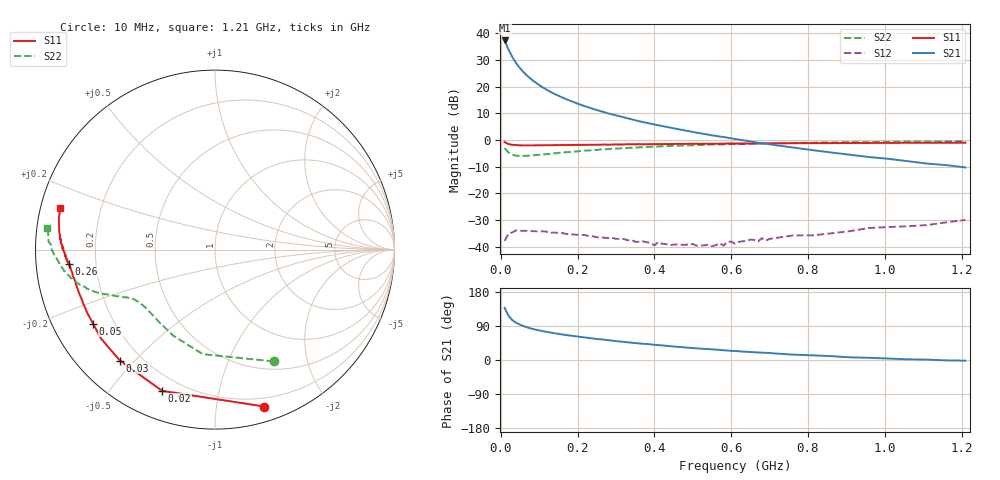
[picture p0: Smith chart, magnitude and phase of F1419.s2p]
! Fri Mar 13 15:57:41 1998
# MHZ  S  MA  R  50.0000
! SCATTERING PARAMETERS :
!  POLYFET RF DEVICES
!  F1419
!  S PARAMETERS
!  VDS=50V, IDQ=400mA
!FREQ  S11MAG S11ANG S21MAG S21ANG S12MAG S12ANG S22MAG S22ANG
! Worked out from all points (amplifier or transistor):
!   81 points, 10 MHz to 1.21 GHz, reference 50 ohm
!   highest |S21| = 37.3 dB at 10 MHz (marker M1)
!   |S21| within 3 dB of that: start of sweep to 18.98 MHz
!   unconditionally stable (mu >= 1): 214.7 MHz to end of sweep
!   at 140 MHz: K = 0.59, MSG = 26.0 dB, |S12| = -34.7 dB
!   at 410 MHz: K = 2.29, MAG = 15.5 dB, |S12| = -38.3 dB
!   at 1.21 GHz: K = 1.35, MAG = 6.3 dB, |S12| = -30.0 dB
!   S11 on the Smith chart (normalised r, x): 10 MHz: 0.12, -1.36; 20 MHz: 0.13, -0.69; 30 MHz: 0.12, -0.45; 50 MHz: 0.12, -0.28; 260 MHz: 0.10, -0.05; 1.21 GHz: 0.06, +0.13
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10  0.9165 -72.5  73.66 137.9  0.01284 49.2  0.7037 -62.3
20  0.8403 -110.6  50.14 116.7  0.01748 29.1  0.5864 -96.7
30  0.8139 -130.6  36.04 105.4  0.01853 20.7  0.5329 -116.0
40  0.8056 -141.9  27.63 98.3  0.02027 15.6  0.5098 -127.4
50  0.795 -148.8  22.3 93.1  0.01988 9.3  0.5033 -134.0
60  0.7942 -153.8  18.53 89.2  0.01983 7.8  0.5031 -138.8
70  0.7933 -157.4  15.78 85.8  0.01979 7.8  0.5075 -142.2
80  0.7928 -160.1  13.68 82.8  0.0196 4.0  0.513 -144.6
90  0.795 -162.2  12.06 80.2  0.01948 4.4  0.521 -146.5
100  0.7959 -163.8  10.75 78.1  0.01923 2.7  0.5272 -148.1
120  0.7991 -166.6  8.745 74.0  0.01908 0.6  0.5451 -150.3
140  0.8013 -168.3  7.336 70.6  0.01842 1.1  0.5635 -151.9
170  0.8047 -170.6  5.853 65.9  0.01737 -2.9  0.5911 -153.8
210  0.8113 -172.5  4.538 60.5  0.01674 -1.8  0.623 -155.8
260  0.8173 -174.6  3.476 54.5  0.01496 0.2  0.6638 -157.9
340  0.8325 -176.5  2.457 45.6  0.0134 5.2  0.7172 -161.1
410  0.8373 -178.7  1.895 39.3  0.0122 16.3  0.756 -164.2
490  0.85 179.4  1.463 32.2  0.01105 28.4  0.7957 -167.0
610  0.8602 177.3  1.045 23.9  0.01139 51.6  0.8418 -171.2
810  0.875 173.0  0.6484 12.4  0.01629 71.5  0.8897 -177.5
1010  0.8856 169.2  0.4441 3.8  0.02336 82.2  0.9281 177.3
1210  0.8927 165.1  0.3065 -1.7  0.03174 83.8  0.944 172.7
